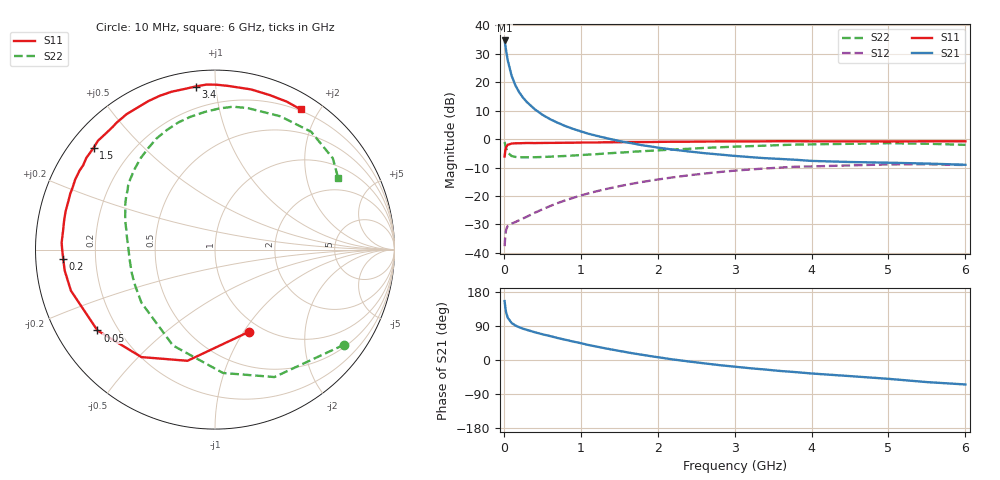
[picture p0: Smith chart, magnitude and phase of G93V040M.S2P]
! SIEMENS Small Signal Semiconductors
! BFG235
! Si NPN RF Bipolar Junction Transistor in SOT223
! VCE = 3 V  IC = 40 mA
! Common Emitter S-Parameters:  July  1994
# GHz  S  MA  R  50
!  f  S11  S21  S12  S22
! GHz  MAG  ANG  MAG  ANG  MAG  ANG  MAG  ANG
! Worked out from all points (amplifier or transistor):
!   40 points, 10 MHz to 6 GHz, reference 50 ohm
!   highest |S21| = 34.7 dB at 10 MHz (marker M1)
!   |S21| within 3 dB of that: start of sweep to 26.69 MHz
!   unconditionally stable (mu >= 1): 524.7 MHz to 1.327 GHz
!   at 200 MHz: K = 0.64, MSG = 22.5 dB, |S12| = -28.5 dB
!   at 1.5 GHz: K = 0.98, MSG = 8.0 dB, |S12| = -16.6 dB
!   at 6 GHz: K = 0.94, MSG = 0.0 dB, |S12| = -9.1 dB
!   S11 on the Smith chart (normalised r, x): 10 MHz: 0.87, -1.05; 50 MHz: 0.13, -0.31; 200 MHz: 0.08, -0.03; 1.5 GHz: 0.07, +0.36; 3.4 GHz: 0.08, +0.88; 6 GHz: 0.18, +1.77
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0.01  0.4957 -67.7  54.43 155.6  0.0131 67.0  0.8939 -36.3
0.02  0.6382 -103.9  44.37 137.6  0.0212 51.5  0.7835 -65.0
0.03  0.7257 -124.4  35.93 125.4  0.0257 41.4  0.6888 -86.3
0.05  0.7949 -145.5  24.57 111.8  0.0297 31.3  0.5833 -113.7
0.1  0.8348 -164.1  13.17 97.9  0.0326 26.9  0.5055 -144.2
0.15  0.8456 -172.1  8.875 91.1  0.0348 29.9  0.4869 -157.4
0.2  0.847 -176.4  6.653 86.5  0.0375 33.4  0.4816 -164.6
0.25  0.8511 -179.7  5.364 82.6  0.0403 36.3  0.4787 -169.5
0.3  0.8554 177.4  4.481 79.5  0.0433 39.3  0.4789 -173.4
0.4  0.8529 172.8  3.373 73.4  0.0505 43.9  0.4806 -178.6
0.5  0.8564 168.8  2.694 68.0  0.0581 47.2  0.485 177.4
0.6  0.8592 165.5  2.248 63.2  0.0664 48.9  0.4914 173.8
0.7  0.8605 161.7  1.941 58.0  0.0751 50.1  0.4987 170.6
0.9  0.8657 156.2  1.516 48.7  0.0927 49.9  0.5146 165.0
1.1  0.8736 149.8  1.244 39.6  0.1111 48.6  0.5345 159.4
1.5  0.883 139.9  0.927 24.0  0.1486 43.1  0.5791 148.5
2.2  0.901 123.2  0.654 1.4  0.2128 29.3  0.657 129.0
3.2  0.9106 101.2  0.483 -21.7  0.2924 5.7  0.7526 100.4
3.4  0.9151 96.8  0.462 -25.2  0.3048 0.7  0.7688 94.3
4.5  0.9148 77.3  0.396 -42.5  0.3449 -25.1  0.8273 63.8
5.5  0.9161 64.2  0.372 -58.3  0.3611 -47.3  0.8307 37.8
6  0.9156 58.5  0.354 -64.6  0.3502 -55.6  0.7936 30.2
